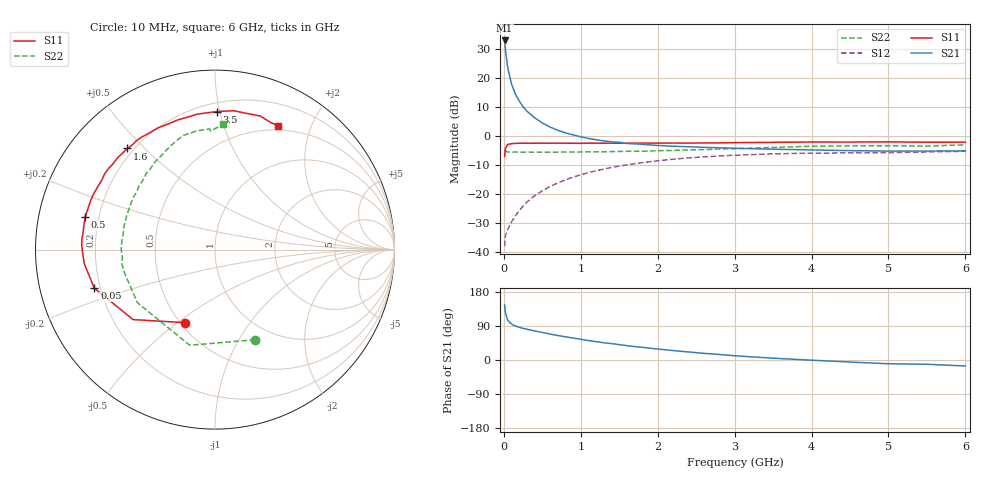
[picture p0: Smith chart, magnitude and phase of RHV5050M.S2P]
! SIEMENS Small Signal Semiconductors
! BFR106
! Si NPN RF Bipolar Junction Transistor in SOT23
! VCE = 0.5 V  IC = 50 mA
! Common Emitter S-Parameters:  August  1996
# GHz  S  MA  R  50
!  f  S11  S21  S12  S22
! GHz  MAG  ANG  MAG  ANG  MAG  ANG  MAG  ANG
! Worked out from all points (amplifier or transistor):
!   36 points, 10 MHz to 6 GHz, reference 50 ohm
!   highest |S21| = 32.9 dB at 10 MHz (marker M1)
!   |S21| within 3 dB of that: start of sweep to 20.26 MHz
!   unconditionally stable (mu >= 1): 99.52 MHz to end of sweep
!   at 250 MHz: K = 1.27, MAG = 14.0 dB, |S12| = -24.3 dB
!   at 1.4 GHz: K = 1.21, MAG = 1.7 dB, |S12| = -11.0 dB
!   at 6 GHz: K = 1.03, MAG = -1.1 dB, |S12| = -5.4 dB
!   S11 on the Smith chart (normalised r, x): 10 MHz: 0.53, -0.53; 50 MHz: 0.18, -0.15; 500 MHz: 0.15, +0.12; 1.6 GHz: 0.18, +0.45; 3.5 GHz: 0.26, +0.98; 6 GHz: 0.45, +1.54
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0.01  0.44 -112.3  44.27 145.0  0.0124 59.0  0.5498 -66.0
0.02  0.6003 -139.5  31.54 125.9  0.0186 46.3  0.5512 -104.8
0.05  0.7056 -162.2  15.08 105.1  0.0241 43.2  0.5238 -145.6
0.1  0.7322 -173.7  7.811 94.7  0.0325 50.4  0.5194 -164.4
0.15  0.7379 -178.7  5.247 89.7  0.0411 57.2  0.5254 -171.1
0.2  0.7426 178.1  3.974 86.2  0.0512 61.4  0.5182 -175.3
0.25  0.7439 175.6  3.169 83.4  0.0611 63.7  0.5211 -178.5
0.3  0.7416 173.4  2.66 81.2  0.0717 65.0  0.5223 179.6
0.4  0.7427 169.1  2.044 76.8  0.0922 66.4  0.5212 176.0
0.5  0.746 165.8  1.668 72.8  0.1124 66.1  0.52 172.9
0.6  0.7436 162.1  1.415 68.6  0.133 65.4  0.5182 170.4
0.7  0.7448 158.5  1.247 64.6  0.153 64.3  0.5219 168.1
0.9  0.7417 152.4  1.036 57.9  0.1934 60.9  0.5226 163.1
1.1  0.7458 145.5  0.899 51.3  0.2303 57.3  0.5275 159.1
1.6  0.7454 130.9  0.736 37.8  0.3147 47.2  0.5388 148.3
2.2  0.749 115.3  0.659 24.9  0.3938 35.3  0.5576 136.1
3  0.761 97.7  0.608 11.2  0.4619 20.9  0.5992 121.1
3.5  0.7691 89.3  0.587 4.8  0.4871 13.4  0.6296 113.1
4.5  0.7791 76.4  0.554 -5.4  0.5061 0.5  0.6691 98.7
5  0.7858 71.3  0.544 -9.9  0.5106 -4.5  0.6733 92.5
5.5  0.7732 66.4  0.545 -11.3  0.5258 -6.9  0.6623 92.1
6  0.7749 62.9  0.549 -15.8  0.5395 -12.8  0.6991 86.2
